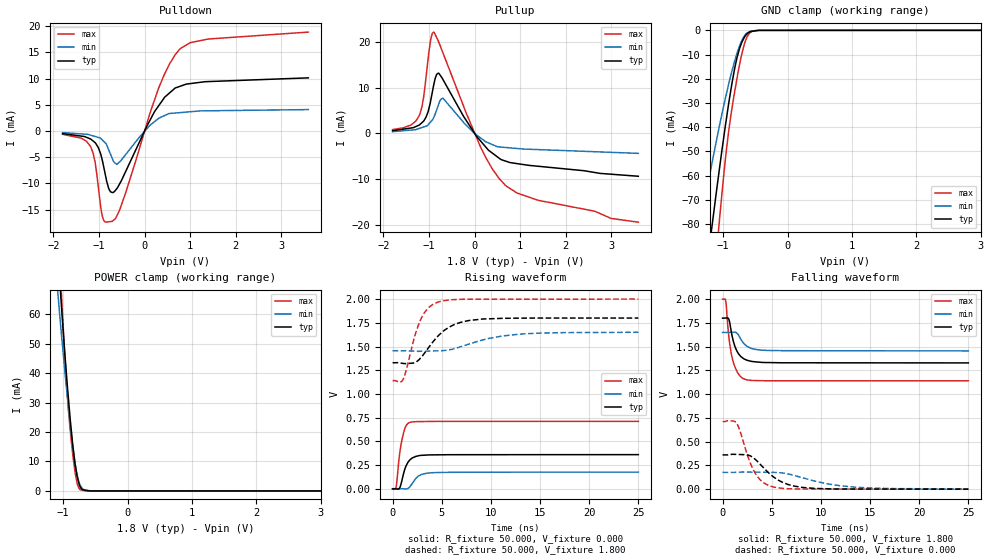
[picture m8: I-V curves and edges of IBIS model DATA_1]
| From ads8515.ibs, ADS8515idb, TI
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|   DATA OUTPUT Model  1.8V
[Model] DATA_1
Model_type 3-state
Polarity   Non-Inverting
Enable   Active-Low
Vmeas = 0.9
Vref = 0.9
Cref = 15pF
Rref = 50
| AVERAGE   typ   min   max
C_comp   1.1393973E-11   1.0101271E-11   1.2147125E-11
| HIGH out
|C_comp   1.2831080E-11   1.1439300E-11   1.3253420E-11
| LOW out
|C_comp   9.9568650E-12   8.7632420E-12   1.1040830E-11
[Voltage Range]   1.8   1.65   2
[Temperature Range]   27   85   -40
[Pullup Reference]   1.8   1.65   2
[Pulldown Reference]   0   0   0
[Power Clamp Reference]   1.8   1.65   2
[GND Clamp Reference]   0   0   0
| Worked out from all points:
|   slope of the pulldown table from 0 to 0.27 V, typ, clamps not added: 62.2 ohm
|   slope of the pullup table from 0 to 0.27 V, typ, clamps not added: 82.5 ohm
|   GND clamp passes 1 mA (typ) near -0.61 V on its own axis
|   POWER clamp passes 1 mA (typ) near -0.72 V on its own axis
|   falling waveform, R_fixture 50.000, V_fixture 1.800: 20-80 % time 831ps typ, 982ps min, 722ps max; typ from 1.8 V to 1.33 V
|   rising waveform, R_fixture 50.000, V_fixture 0.000: 20-80 % time 713ps typ, 887ps min, 573ps max; typ from 0 V to 0.361 V
|   rising waveform, R_fixture 50.000, V_fixture 1.800: 20-80 % time 2.6ns typ, 4.38ns min, 1.54ns max; typ from 1.33 V to 1.8 V
|   falling waveform, R_fixture 50.000, V_fixture 0.000: 20-80 % time 2.51ns typ, 4.51ns min, 1.57ns max; typ from 0.361 V to 0 V
[Pulldown]
|   Voltage   I  typ   I  min   I  max
-1.8V     -493.3uA   -302.1uA   -631.6uA
-1.192V   -1.502mA   -772.2uA   -2.87mA
-1.086V   -2.222mA   -1.042mA   -5.974mA
-965.5mV  -4.335mA   -1.375mA   -14.33mA
-916.2mV  -6.038mA   -1.808mA   -16.61mA
-790mV    -10.91mA   -3.544mA   -17.33mA
-714.5mV  -11.71mA   -5.132mA   -17.25mA
-597.2mV  -10.87mA   -6.298mA   -15.99mA
320.6mV   4.96mA     2.479mA    8.443mA
783.7mV   8.549mA    3.514mA    15.73mA
1.391V    9.433mA    3.86mA     17.55mA
3.595V    10.14mA    4.088mA    18.88mA
[GND Clamp]
|   Voltage   I  typ   I  min   I  max
-1.8V     -223.4mA   -151.4mA   -315.8mA
-1.353V   -119.8mA   -80.47mA   -170mA
-1.173V   -80.86mA   -54.79mA   -113.3mA
-1.072V   -60.03mA   -41.23mA   -82.66mA
-1.049V   -55.37mA   -38.29mA   -75.78mA
-949.6mV  -36.54mA   -26.2mA    -49.4mA
-878.2mV  -24.29mA   -18.32mA   -34.8mA
-748.4mV  -7.761mA   -6.725mA   -14.66mA
-641.1mV  -1.806mA   -1.336mA   -3.489mA
-562.1mV  -454.4uA   -292.1uA   -579.3uA
-453.3mV  -20.52uA   -42.8uA    -21.93uA
3.595V    0A         0A         0A
[Pullup]
|   Voltage   I  typ   I  min   I  max
-1.8V     604.7uA    404.2uA    846.7uA
-1.21V    1.88mA     1.113mA    4.004mA
-1.12V    2.673mA    1.415mA    7.785mA
-1.02V    4.761mA    1.904mA    16.27mA
-961.4mV  7.229mA    2.549mA    20.53mA
-897.5mV  10.54mA    3.473mA    22.07mA
-796.5mV  13.14mA    6.123mA    20.14mA
-689mV    11.65mA    7.636mA    17.42mA
133mV     -1.637mA   -976.6uA   -2.971mA
673.8mV   -5.985mA   -3.035mA   -11.26mA
1.383V    -7.117mA   -3.498mA   -14.5mA
3.595V    -9.306mA   -4.323mA   -19.3mA
[POWER Clamp]
|   Voltage   I  typ   I  min   I  max
-1.8V     370.3mA    302mA      454.1mA
-1.078V   80.13mA    66.12mA    90mA
-1.039V   66.9mA     56.23mA    72.31mA
-1.031V   64.15mA    54.19mA    68.82mA
-1.009V   57.45mA    49.11mA    59.64mA
-949.6mV  39.81mA    35.22mA    37.08mA
-885.4mV  23.18mA    21.61mA    19.45mA
-812.7mV  8.802mA    9.097mA    6.023mA
-778.2mV  4.554mA    4.992mA    2.243mA
-738.5mV  1.544mA    2.079mA    452.7uA
-577.5mV  14.63uA    16.97uA    12.92uA
3.595V    0A         0A         0A
[Ramp]
R_load = 50
|   typ   min   max
dV/dt_r   0.216437/7.10384e-010  0.106791/8.75832e-010  0.426816/5.70844e-010
dV/dt_f   0.28237/8.23906e-010  0.116758/9.54136e-010  0.515708/7.19303e-010
[Falling Waveform]
R_fixture = 50.000
V_fixture = 1.800
V_fixture_min = 1.650
V_fixture_max = 2.000
C_fixture = 0.000
|  time   V  typ   V  min   V  max
0s        1.8V       1.65V      2V
327.7ps   1.802V     1.65V      1.978V
527.8ps   1.802V     1.65V      1.723V
683.6ps   1.773V     1.65V      1.565V
864.8ps   1.671V     1.651V     1.439V
1.082ns   1.563V     1.652V     1.341V
1.614ns   1.426V     1.623V     1.213V
2.343ns   1.364V     1.516V     1.154V
4.381ns   1.333V     1.461V     1.141V
25ns      1.329V     1.455V     1.14V
[Rising Waveform]
R_fixture = 50.000
V_fixture = 0.000
V_fixture_min = 0.000
V_fixture_max = 0.000
C_fixture = 0.000
|  time   V  typ   V  min   V  max
0s        405.5nV    2.069mV    1.305uV
287.3ps   99.11uV    2.086mV    -2.658mV
357.6ps   123.2uV    2.09mV     16.7mV
758.4ps   16.93mV    2.114mV    398.9mV
1.149ns   172.6mV    522uV      601.8mV
1.429ns   253.4mV    -129.2uV   674.1mV
1.812ns   309.9mV    29.56mV    702.1mV
2.667ns   349.2mV    137.1mV    709mV
4.017ns   358.1mV    170.3mV    710.7mV
25ns      360.7mV    176.7mV    711.4mV
[Rising Waveform]
R_fixture = 50.000
V_fixture = 1.800
V_fixture_min = 1.650
V_fixture_max = 2.000
C_fixture = 0.000
|  time   V  typ   V  min   V  max
0s        1.329V     1.455V     1.14V
1.042ns   1.322V     1.455V     1.148V
2.288ns   1.332V     1.451V     1.619V
2.839ns   1.378V     1.45V      1.779V
3.621ns   1.482V     1.452V     1.904V
4.628ns   1.611V     1.454V     1.968V
6.296ns   1.732V     1.478V     1.994V
9.172ns   1.79V      1.569V     1.999V
14.61ns   1.8V       1.64V      1.999V
25ns      1.8V       1.65V      2V
[Falling Waveform]
R_fixture = 50.000
V_fixture = 0.000
V_fixture_min = 0.000
V_fixture_max = 0.000
C_fixture = 0.000
|  time   V  typ   V  min   V  max
0s        360.7mV    176.7mV    711.4mV
1.401ns   366mV      177.6mV    698.4mV
2.694ns   355.4mV    180.1mV    308.7mV
3.249ns   320.1mV    179.5mV    180.4mV
4.032ns   239.7mV    178.6mV    79.58mV
5.036ns   140.7mV    177.4mV    26.98mV
6.691ns   48.41mV    159.4mV    4.716mV
9.415ns   7.51mV     84.51mV    1.176mV
13.81ns   1.528mV    18.69mV    844.6uV
25ns      405.5nV    2.069mV    1.305uV
